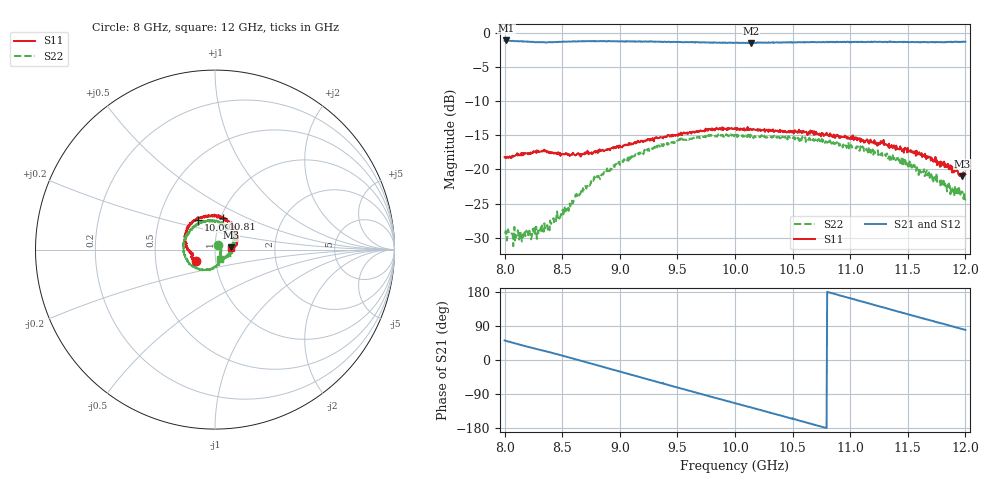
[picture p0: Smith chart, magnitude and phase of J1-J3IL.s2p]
!Agilent Technologies,N5230C,MY49001174,A.09.42.21
!Agilent N5230C: A.09.42.21
!Date: Saturday, January 30, 2016 08:41:00
!Correction: S11(Full 2 Port(1,2))
!S21(Full 2 Port(1,2))
!S12(Full 2 Port(1,2))
!S22(Full 2 Port(1,2))
!S2P File: Measurements: S11, S21, S12, S22:
# Hz S  dB  R 50
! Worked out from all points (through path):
!   801 points, 8 GHz to 12 GHz, reference 50 ohm
!   highest |S21| = -1.13 dB at 8.015 GHz (marker M1); lowest = -1.5 dB at 10.14 GHz (marker M2)
!   group delay of S21, straight-line fit = 231 ps
!   lowest |S11| = -20.9 dB at 11.97 GHz (marker M3), VSWR 1.20, Z = 59.7 + j1.52 ohm
!   |S11| at or under -10 dB: start of sweep to end of sweep
!   |S22| runs from -31.2 to -14.9 dB; largest |S21 - S12| = 0.015
!   S11 on the Smith chart (normalised r, x): 8 GHz: 0.80, -0.11; 10.09 GHz: 0.78, +0.27; 10.81 GHz: 1.03, +0.37; 12 GHz: 1.20, +0.02
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8e9  -18.19 -148.1  -1.17 51.7  -1.14 51.6  -29.36 56.2
8.015e9  -18.20 -147.2  -1.13 50.4  -1.15 50.4  -29.27 52.2
8.145e9  -17.58 -151.0  -1.25 39.5  -1.28 39.4  -29.97 8.8
8.37e9  -17.34 -164.1  -1.42 21.9  -1.37 22.2  -28.13 -39.8
8.67e9  -17.82 -170.3  -1.25 -2.5  -1.24 -2.6  -23.37 -66.1
8.97e9  -16.67 -178.1  -1.24 -27.9  -1.24 -27.9  -19.22 -100.4
9.155e9  -15.80 175.6  -1.29 -43.5  -1.29 -43.4  -17.63 -117.4
9.335e9  -15.41 165.8  -1.32 -58.7  -1.31 -58.7  -16.50 -136.1
9.54e9  -14.98 155.8  -1.38 -75.9  -1.33 -75.8  -15.48 -157.2
9.685e9  -14.54 146.6  -1.39 -88.1  -1.38 -88.0  -15.35 -169.7
1e10  -13.96 126.3  -1.48 -114.0  -1.48 -114.0  -14.98 160.9
1.0085e10  -14.30 119.8  -1.48 -121.0  -1.47 -120.7  -14.95 152.4
1.014e10  -14.12 116.5  -1.52 -125.4  -1.45 -125.3  -15.24 148.8
1.0435e10  -14.38 98.9  -1.41 -149.8  -1.42 -149.8  -15.23 124.4
1.067e10  -14.65 84.6  -1.36 -169.4  -1.40 -169.0  -15.42 103.5
1.0815e10  -14.92 75.4  -1.36 178.6  -1.37 178.7  -15.87 90.4
1.1095e10  -15.52 54.7  -1.36 154.9  -1.31 155.1  -17.06 64.0
1.1335e10  -16.22 39.9  -1.34 134.8  -1.36 134.7  -18.14 35.2
1.164e10  -17.86 19.5  -1.34 108.9  -1.41 109.4  -19.97 -2.1
1.181e10  -19.33 11.7  -1.40 95.4  -1.34 95.1  -21.63 -30.7
1.197e10  -20.95 8.1  -1.33 81.7  -1.32 81.9  -23.21 -60.0
1.2e10  -20.74 5.7  -1.30 79.4  -1.33 79.3  -24.52 -64.6
